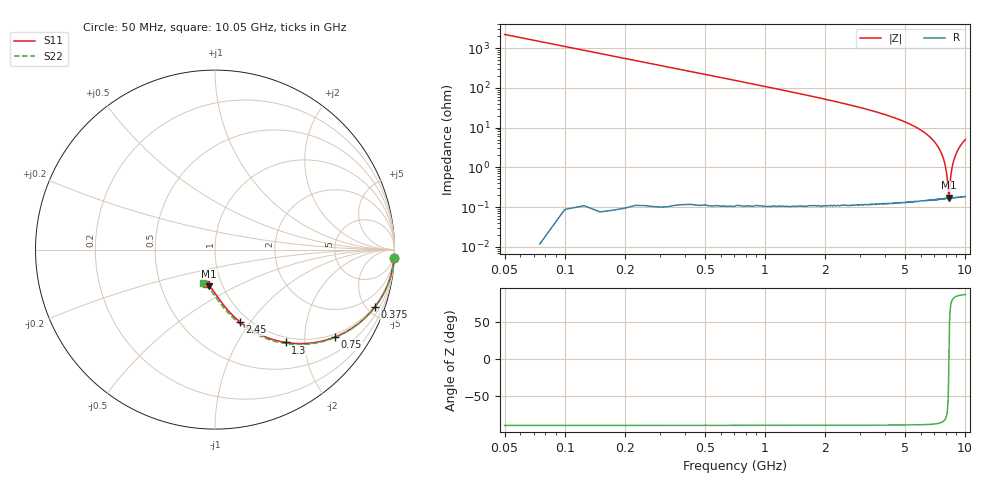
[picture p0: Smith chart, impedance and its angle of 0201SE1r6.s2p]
! AVX Thin Film Operation		Date: August 2001
! Description: Accu-P® Series, Thin Film, SMD, RF Capacitor
! Part Number: 02013J1R6ABW
! 50 MHz  -  10.05 GHz
! Serial Measurements
# mhz S db R 50
!	S11		S21		S12		S22
!	dB	Phase	dB	Phase	dB	Phase	dB	Phase
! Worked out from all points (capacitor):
!   401 points, 50 MHz to 10.05 GHz, reference 50 ohm
!   read as one part in series: C = 1.45 pF near 100 MHz
!   lowest |Z| = 172 mohm at 8.325 GHz (marker M1)
!   series resonance near 8.31 GHz, so ESL is about 250 pH
!   S11 on the Smith chart (normalised r, x): 50 MHz: 1, -42; 375 MHz: 0.91, -5.59; 750 MHz: 0.91, -2.81; 1.3 GHz: 0.91, -1.63; 2.45 GHz: 0.91, -0.89; 10.05 GHz: 0.85, -0.34
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50  -0.01 -2.7  -26.86 87.3  -26.86 87.3  -0.01 -2.8
75  -0.02 -4.1  -23.34 85.9  -23.34 85.9  -0.02 -4.1
125  -0.06 -6.8  -18.94 83.2  -18.94 83.2  -0.06 -6.9
150  -0.08 -8.2  -17.39 81.8  -17.39 81.8  -0.08 -8.2
200  -0.14 -10.8  -14.95 79.1  -14.95 79.1  -0.14 -10.9
275  -0.26 -14.7  -12.31 75.2  -12.31 75.2  -0.26 -14.9
375  -0.48 -19.8  -9.83 70.1  -9.83 70.1  -0.48 -20.0
450  -0.67 -23.4  -8.45 66.5  -8.45 66.5  -0.67 -23.6
550  -0.97 -27.9  -7.01 61.9  -7.01 61.9  -0.97 -28.2
750  -1.65 -36.1  -5.01 53.7  -5.01 53.7  -1.65 -36.5
1000  -2.59 -44.6  -3.49 45.1  -3.49 45.1  -2.59 -45.1
1300  -3.73 -52.7  -2.40 36.9  -2.40 36.9  -3.73 -53.4
1725  -5.24 -61.2  -1.55 28.2  -1.55 28.2  -5.24 -62.1
2075  -6.35 -66.5  -1.15 22.9  -1.15 22.9  -6.35 -67.6
2450  -7.40 -70.9  -0.88 18.3  -0.88 18.3  -7.40 -72.3
3400  -9.51 -79.0  -0.53 9.9  -0.53 9.9  -9.51 -80.9
4175  -10.77 -83.7  -0.39 4.9  -0.39 4.9  -10.77 -86.0
5050  -11.83 -87.9  -0.31 0.5  -0.31 0.5  -11.84 -90.6
6725  -13.12 -94.3  -0.23 -6.4  -0.23 -6.4  -13.13 -97.8
8325  -13.76 -99.3  -0.20 -11.9  -0.20 -11.9  -13.78 -103.5
8400  -13.78 -99.5  -0.20 -12.1  -0.20 -12.1  -13.80 -103.8
10050  -14.06 -104.2  -0.19 -17.2  -0.19 -17.2  -14.09 -109.2
